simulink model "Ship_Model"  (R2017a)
settings: Solver=VariableStepAuto  StartTime=0.0  StopTime=10  FixedStep=1  RelTol=1e-3

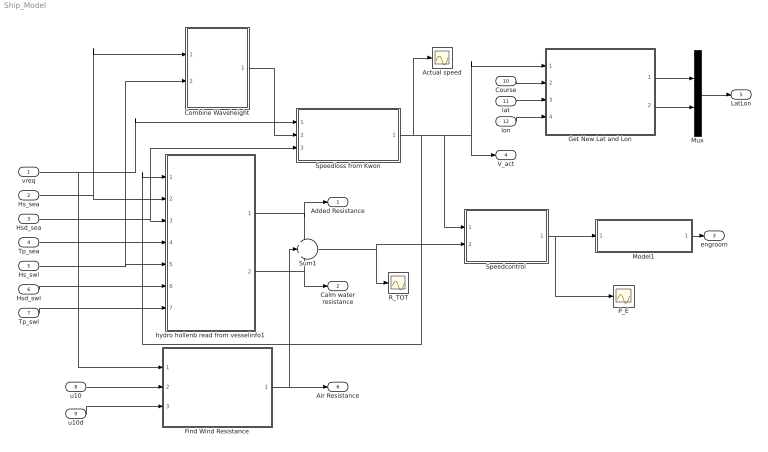
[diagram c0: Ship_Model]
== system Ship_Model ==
  vreq : Inport
  Hs_sea : Inport  Port=2
  Hsd_sea : Inport  Port=3
  Tp_sea : Inport  Port=4
  Hs_swl : Inport  Port=5
  Hsd_swl : Inport  Port=6
  Tp_swl : Inport  Port=7
  u10 : Inport  Port=8
  u10d : Inport  Port=9
  Course : Inport  Port=10
  lat : Inport  Port=11
  lon : Inport  Port=12
  Actual speed : Scope
  Combine Waveheight : ModelReference  ModelNameDialog=Combine_Waveheight  SimulationMode=Normal  ModelReferenceVersion=1.3
  Find Wind Resistance : ModelReference  ModelNameDialog=Wind_Resistance_Model.slx  SimulationMode=Normal  ModelReferenceVersion=1.5
  Get New Lat and Lon : ModelReference  ModelNameDialog=getLatLon  SimulationMode=Normal  ModelReferenceVersion=1.5
  Model1 : ModelReference  ModelNameDialog=EngRoomONE  SimulationMode=Normal  ModelReferenceVersion=1.56
  Mux : Mux  Inputs=2
  P_E : Scope
  R_TOT : Scope
  Speedcontrol : ModelReference  ModelNameDialog=speedcontrol.slx  SimulationMode=Normal  ModelReferenceVersion=1.22
  Speedloss from Kwon : ModelReference  ModelNameDialog=Kwon_speed_loss  SimulationMode=Normal  ModelReferenceVersion=1.21
  Sum1 : Sum  Inputs=+++
  hydro hollenb read from vesselinfo1 : ModelReference  ModelNameDialog=hydroHollenbach  SimulationMode=Normal  ModelReferenceVersion=1.60
  Added Resistance : Outport
  Calm water resistance : Outport  Port=2
  engroom : Outport  Port=3
  V_act : Outport  Port=4
  LatLon : Outport  Port=5
  Air Resistance : Outport  Port=6
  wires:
  Tp_swl/1 -> hydro hollenb read from vesselinfo1/7
  Hsd_swl/1 -> hydro hollenb read from vesselinfo1/6
  Hs_swl/1 -> hydro hollenb read from vesselinfo1/5, Combine Waveheight/2
  Tp_sea/1 -> hydro hollenb read from vesselinfo1/4
  Hsd_sea/1 -> hydro hollenb read from vesselinfo1/3, Speedloss from Kwon/3
  Hs_sea/1 -> hydro hollenb read from vesselinfo1/2, Combine Waveheight/1
  vreq/1 -> Find Wind Resistance/1, Speedloss from Kwon/1
  hydro hollenb read from vesselinfo1/1 -> Sum1/1, Added Resistance/1
  hydro hollenb read from vesselinfo1/2 -> Sum1/3, Calm water resistance/1
  Sum1/1 -> R_TOT/1, Speedcontrol/2
  Speedcontrol/1 -> P_E/1, Model1/1
  Speedloss from Kwon/1 -> hydro hollenb read from vesselinfo1/1, Get New Lat and Lon/1, V_act/1, Speedcontrol/1, Actual speed/1
  Course/1 -> Get New Lat and Lon/2
  lat/1 -> Get New Lat and Lon/3
  lon/1 -> Get New Lat and Lon/4
  Get New Lat and Lon/1 -> Mux/1
  Get New Lat and Lon/2 -> Mux/2
  Mux/1 -> LatLon/1
  Combine Waveheight/1 -> Speedloss from Kwon/2
  u10d/1 -> Find Wind Resistance/3
  u10/1 -> Find Wind Resistance/2
  Find Wind Resistance/1 -> Sum1/2, Air Resistance/1
  Model1/1 -> engroom/1
